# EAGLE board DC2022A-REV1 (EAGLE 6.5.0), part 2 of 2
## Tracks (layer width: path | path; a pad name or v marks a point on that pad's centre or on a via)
+3V3  (via drill 0.25)
  Top 0.203: R23.1 46.14,5.12 45.85,4.83 44.07,4.83 44.07,7.49 43.84,7.47 R16.R1_2 | U6.8 44.03,12.99 44.07,12.95 v43.18,12.95 | 50.93,11.81 U9.18 | R17.1 56.13,7.87 56.13,7.37 55.88,7.11 54.48,7.11 54.23,7.37 54.23,10.67 53.59,11.3 53.59,12.19 | C18.2 27.29,22.25
  Top 0.305: U6.8 44.32,12.95 44.32,11.94 44.3,11.92 44,11.92 C22.1 R16.R4_2 | U4.12 U4.11 29.41,22.42 29.34,22.35 v28.45,22.35 28.45,21.84 C18.2
  Top 0.406: R16.R1_2 R16.R2_2 R16.R3_2 R16.R4_2 | 50.93,11.81 51.31,12.19 53.59,12.19 53.59,12.83 v53.85,13.08 | v28.45,22.35 28.45,22.28 | R15.R1_2 R15.R2_2 R15.R3_2 R15.R4_2 41.62,18.2 41.36,18.2 41.27,18.29 v41.27,19.05
  Route15 0.406: v53.85,13.08 53.85,12.7 53.47,12.32 52.32,12.32 51.94,11.94 45.31,11.94 U6.8 43.22,12.99 v43.18,12.95
  Bottom 0.203: R39.1 R37.1 53.17,15.28 53.85,14.61 v53.85,13.08 | R44.1 23.07,29.21
  Bottom 0.406: v43.18,12.95 43.18,13.59 41.53,15.24 40.83,15.24 R38.R1_2 R38.R2_2 R38.R3_2 R38.R4_2 40.73,18.92 | U12.5 19.81,27.05 19.56,27.3 19.56,29.21 C50.1 23.07,29.21 | 40.73,18.92 40.73,20.23 40.26,20.57 36.83,20.57 35.81,19.56 35.69,19.43 29.97,19.43 29.46,19.94 23.11,19.94 22.35,20.7 22.35,22.1 23.16,22.1 | v41.27,19.05 40.85,19.05 40.73,18.92 | R42.2 23.33,23.91 | 24.38,22.1 28.45,22.1 v28.45,22.35 | R42.2 23.37,24 | 24.38,22.1 24.38,28.83 24.26,28.96 23.41,28.96 R44.1 | 23.16,22.1 23.24,22.1 | 23.24,22.1 23.2,22.19 | 23.2,22.19 23.2,23.88 R42.2 | 23.24,22.1 24.38,22.1 | 23.16,22.1 23.2,22.19
+12V
  Route15 1.016: JP2.14 JP2.13
  pour Top (no thermals): 48.13,30.3 48.13,32.77 57.15,32.77 58.17,33.78 60.58,33.78 61.85,32.64 61.85,30.23 60.33,28.7 53.09,28.7 53.09,29.59 52.32,30.35 50.04,30.35
  pour Bottom (no thermals): 55.12,26.42 55.12,36.45 55.75,37.08 55.75,41.78 56.13,42.16 57.91,42.16 58.29,41.78 58.29,34.29 58.67,33.91 60.58,33.91 61.72,32.89 61.72,30.1 60.07,28.45 60.07,21.08 57.53,18.54 57.53,3.81 57.02,3.3 54.86,3.3 54.86,23.88 57.15,23.88 57.15,26.42
A0_MUX  (via drill 0.25)
  Top 0.203: U9.3 47.88,8.76 47.45,8.38 47.3,8.38 v47.3,8.46 47.3,8.41 47.27,8.38 46.84,8.38 | 46.84,8.38 R16.R2_1 46.59,8.36 46.61,8.38 46.84,8.38
  Bottom 0.203: v47.3,8.46 47.3,8.41 47.27,8.38 46.48,8.38 45.97,7.87 JP3.6
A1_MUX  (via drill 0.25)
  Top 0.203: U9.2 48.67,9.27 47.93,9.27 47.78,9.16 R16.R3_1 46.12,9.16 46.1,9.14 47.3,9.14 | 47.3,9.14 47.4,9.16 | 47.3,9.14 v47.3,9.45 47.3,9.27
  Bottom 0.203: v47.3,9.45 46.41,9.45 46.1,9.14 JP3.7
A2_MUX  (via drill 0.25)
  Top 0.203: 47.3,10.16 48.39,10.16 48.39,9.78 48.64,9.78 U9.1 | R16.R4_1 46.44,10.12 46.48,10.16 47.3,10.16 | 47.3,10.16 v47.3,10.54
  Bottom 0.203: v47.3,10.54 45.21,10.54 JP3.8
ALERTB  (via drill 0.25)
  Top 0.203: U4.31 37.16,18.72 37.34,18.54 37.85,18.54 38.35,18.03 38.35,15.37 38.86,14.86 39.62,14.86 | v42.93,16.51 42.93,15.24 42.55,14.86 39.62,14.86 | R15.R4_1 39.62,15.62 39.62,14.86
  Route15 0.203: v30.73,29.97 30.73,29.34 31.11,28.96 32.51,28.96 32.77,29.21 32.77,30.73 33.02,30.99 33.66,30.99 34.16,31.5 39.12,31.5 39.75,30.86 41.91,30.86 42.16,30.61 42.16,30.1 43.05,29.21 v43.05,28.83
  Bottom 0.203: JP1.3 46.55,38.42 46.23,38.1 45.09,38.1 43.56,36.58 43.56,33.78 43.31,33.53 43.31,28.83 | 43.31,28.83 43.31,20.83 44.2,19.94 44.2,16.51 | 44.2,16.51 44.2,14.73 44.7,14.22 44.7,12.19 44.96,11.94 46.99,11.94 48.13,10.79 48.13,8.26 46.48,6.6 46.48,3.78 JP2.3 | TP12.TP 12.06,26.92 12.57,26.42 16.13,26.42 | 44.2,16.51 v42.93,16.51 | U12.1 18.3,26.4 18.29,26.42 16.13,26.42 | 16.13,26.42 16.13,29.72 16.89,30.48 24.89,30.48 25.27,30.1 30.61,30.1 v30.73,29.97 | v43.05,28.83 43.31,28.83
CTRL  (via drill 0.25)
  Top 0.203: C28.1 55.24,10.03 55.63,10.41 57.02,10.41 57.28,10.67 S1.5 | U4.32 37.65,19.38 37.72,19.43 37.97,19.43 38.41,19.87 U4.33 39.37,20.13 | U4.22 U4.23 33.16,18.81 32.77,18.41 30.99,18.41 30.35,17.78 28.57,17.78 v28.57,17.65 | 39.37,20.13 v39.37,19.81 39.37,18.23 R15.R1_1 | 39.37,20.13 41.98,20.13 v43.18,18.92
  Top 0.406: S1.5 S1.2
  Route15 0.203: v43.18,18.92 43.31,18.92 43.81,18.41 43.81,17.02 44.96,15.88 45.97,15.88 48.01,13.84 50.55,13.84 51.94,15.24 53.21,15.24 54.86,13.59 55.5,13.59 57.15,11.94 S1.5
  Bottom 0.203: 42.55,18.92 42.55,27.56 42.04,28.07 42.04,29.59 42.55,30.1 42.55,34.04 42.8,34.29 42.8,37.08 43.43,37.72 43.43,41.15 | JP2.2 44.55,1.65 43.69,1.65 43.43,1.91 43.43,4.83 43.56,4.95 43.56,12.06 43.94,12.45 43.94,13.72 41.78,15.88 41.78,18.41 42.29,18.92 42.55,18.92 | 43.43,41.15 44.55,41.15 JP1.2 | R56.2 43.43,43.56 43.43,41.15 | 42.55,18.92 v43.18,18.92 | v28.57,17.65 28.32,17.65 27.81,18.16 27.81,18.8 28.19,19.18 29.34,19.18 29.59,18.92 35.94,18.92 36.96,19.94 39.37,19.94 v39.37,19.81
CTRL_P
  Bottom 0.203: R56.1 45.68,43.22 45.72,43.18 50.55,43.18 51.54,42.19 51.54,38.38 52.83,37.08 TP6.TP
DACP_CH0  (via drill 0.25)
  Top 0.203: v36.07,29.46 35.94,29.46 35.69,29.21 35.69,28.4 U4.53
  Route15 0.203: v25.02,16.64 26.16,17.78 26.16,28.32 26.8,28.96 v27.18,28.96
  Bottom 0.203: R36.2 17.02,12.45 17.27,12.45 | TP28.1 17.27,14.73 18.16,15.62 24.64,15.62 25.02,16 v25.02,16.64 | v27.18,28.96 26.92,28.7 26.92,24.13 27.43,23.11 33.53,23.11 35.05,24.51 35.05,26.16 35.56,26.54 35.56,29.34 35.69,29.46 v36.07,29.46
  Bottom 0.406: 17.27,12.45 TP28.1
DACP_CH1  (via drill 0.25)
  Top 0.203: TP24.1 32.64,15.24 32.26,15.62 v32.26,17.78 | U4.54 35.16,29.06 35.31,29.21 35.31,29.59 v36.07,30.35
  Route15 0.203: v32.26,17.78 32.64,17.78 33.53,18.67 33.53,23.62 35.05,25.4 35.05,29.34 v36.07,30.35
  Bottom 0.203: R34.2 32.38,12.45 32.64,12.45
  Bottom 0.406: 32.64,12.45 TP24.1
DACP_CH2
  Top 0.203: TP37.1 21.72,31.5 22.1,31.11 32.38,31.11 32.51,31.11 32.77,30.86 32.77,29.84 33.66,28.96 U4.57
  Bottom 0.203: R48.2 21.97,33.91 21.72,33.91
  Bottom 0.406: TP37.1 21.72,33.91
DACP_CH3  (via drill 0.25)
  Top 0.203: U4.58 33.16,28.44 33.15,28.45 33.15,28.91 32.46,29.59 v32.05,29.59
  Route15 0.203: TP33.1 37.08,32.77 36.83,33.02 36.7,33.02 34.42,33.02 34.04,32.64 34.04,32 33.53,31.5 32.89,31.5 32.13,30.73 32.13,29.67 v32.05,29.59
  Bottom 0.203: R46.2 37.34,33.91 37.08,33.91
  Bottom 0.406: TP33.1 37.08,33.91
EESCL
  Top 0.203: 61.98,6.1 61.72,6.35 R20.1 62.53,6.35 | U10.1 62.32,1.59 62.53,1.78 62.53,6.35 | 62.53,6.35 62.53,6.66 63.12,7.24 63.12,8 63.37,8.26 68.17,8.26 68.67,8.76 68.67,10.29 68.23,10.73 66.52,10.73 J2.11 65.59,9.65
EESDA
  Top 0.203: 61.72,3.43 U10.3 61.72,4.83 R24.1 60.83,4.83 60.83,7.06 60.96,7.19 62.46,7.19 62.61,7.34 62.61,8.26 62.99,8.64 67.41,8.64 67.69,8.89 67.69,9.65 J2.12
EEVCC  (via drill 0.25)
  Top 0.203: 63.32,20.77 62.7,20.77 C19.1
  Top 0.254: U5.8 U5.7
  Top 0.406: R24.2 R20.2 59.94,6.35 | U10.4 58.86,3.49 59.18,3.56 | 59.18,4.79 R24.2 | 59.18,3.56 59.05,3.56 | 59.18,4.79 59.18,4.83 | 59.18,3.56 59.18,4.79 | R24.2 59.18,4.83 | 59.18,4.83 v58.8,4.83 | 59.94,6.35 59.86,6.35 | 59.94,6.35 59.94,7.87 C27.1
  Top 0.813: 68.42,37.85 68.4,37.82 68.58,37.82 68.58,22.48 68.45,22.48 68.4,22.55
  Top 1.016: 68.42,37.85 67.41,38.86 64.14,38.86 63.37,39.62 59.31,39.62 58.04,40.89 58.04,42.55 57.66,42.93 51.05,42.93 50.53,42.4 50.53,41.15 JP1.8 | 64.14,22.48 68.45,22.48 | 64.14,22.48 v64.14,21.84 64.14,21.59 63.32,20.77 U5.8 | 64.14,22.48 v64.14,22.99
  Route15 0.406: v52.58,19.56 54.1,19.56 56.39,21.84 v64.14,21.84
  Bottom 0.406: D1.2 53.48,19.8 53.09,19.56 v52.58,19.56
  Bottom 0.813: J2.1 65.52,19.7 65.5,19.68 64.1,19.68 arc60 64.14,19.81 v64.14,21.84 v64.14,22.99
  pour Bottom (no thermals): 49.78,2.92 57.28,2.92 58.04,3.68 58.04,18.29 60.58,20.83 66.39,20.83 66.39,18.92 62.23,18.92 59.82,16.51 59.82,0.76 49.78,0.76
  pour Top (no thermals): 60.2,21.46 63.12,21.46 63.5,21.84 63.5,23.5 64.9,23.5 64.9,21.72 63.37,20.19 60.2,20.19
FAULTB  (via drill 0.25)
  Top 0.203: U4.25 U4.26 34.47,19.38 34.42,19.3 34.42,17.27 34.8,16.89 v34.8,15.24 | TP7.TP 9.27,31.37 10.16,30.48 14.73,30.48 15.37,29.84 15.37,27.94 15.61,27.7 v17.13,27.7
  Route15 0.203: v43.18,19.81 42.8,19.81 42.29,19.3 42.29,16.13 41.66,15.49 35.05,15.49 v34.8,15.24
  Bottom 0.203: JP2.1 44.29,3.72 44.2,3.81 44.2,6.35 44.07,6.48 44.07,11.94 44.32,12.19 44.32,13.97 42.29,16 42.29,17.65 42.67,18.03 43.43,18.03 43.81,18.41 43.81,19.43 43.43,19.81 v43.18,19.81 42.93,19.81 42.93,27.81 42.42,28.32 42.42,29.34 42.93,29.84 42.93,33.78 43.18,34.04 43.18,36.83 44.58,38.23 44.58,39.13 JP1.1 | v17.13,27.7 U12.3 19.05,27.7 19.05,26.16 19.3,25.91 20.7,25.91 20.95,25.65 20.95,25.02 21.84,24.13 21.84,20.32 22.86,19.3 26.04,19.3 29.72,15.62 32.89,15.62 33.78,14.73 34.29,14.73 v34.8,15.24 35.05,15.49 37.34,15.49 38.08,16.24 R38.R2_1
FB_LTC3604
  Top 0.203: 51.73,23.75 R8.2 51.85,24.42 52.07,24.64 52.7,24.64 52.96,24.89 52.96,27.05 52.7,27.3 52.7,28.96 52.3,29.44 U3.11
  Top 0.305: R9.1 C17.1 51.73,23.75 | R8.2 C13.2
GND  (via drill 0.25, 0.25 pad 0.56)
  Top 0.203: v40.77,13.72 v41.78,13.72 | C24.2 v40.77,13.72 | v40.77,13.72 v39.75,13.72 | v40.77,13.72 40.77,12.2 | R22.1 33.62,6.39 33.53,6.1 | v25.4,13.72 v26.42,13.72 | C23.2 v25.4,13.72 | v25.4,13.72 v24.38,13.72 | v25.4,13.72 25.4,12.2 | R21.1 18.25,6.39 18.16,6.1 | v12.57,32.64 v13.59,32.64 | v13.59,32.64 C9.2 | v13.59,32.64 v14.61,32.64 | v13.59,32.64 13.59,34.16 | R3.1 20.74,39.97 20.83,40.26 | v27.94,32.64 v28.96,32.64 | v28.96,32.64 C10.2 | v28.96,32.64 v29.97,32.64 | v28.96,32.64 28.96,34.16 | R4.1 36.11,39.97 36.2,40.26
  Top 0.305: LED3.N 45.6,17.03 45.85,17.27 45.85,19.43 46.1,19.68 v46.61,19.68
  Top 0.406: 33.53,6.1 33.66,6.22 33.91,6.22 | v34.67,6.22 33.62,6.22 R22.1 | 18.16,6.1 18.29,6.22 18.54,6.22 | v19.3,6.22 18.25,6.22 R21.1 | 20.83,40.26 20.7,40.13 20.45,40.13 | v19.68,40.13 20.74,40.13 R3.1 | 36.2,40.26 36.07,40.13 35.81,40.13 | v35.05,40.13 36.11,40.13 R4.1
  Bottom 0.203: 42.16,3.03 Q5.2 | 42.16,3.03 42.16,3.05 | v42.16,2.29 42.16,3.03 | 26.8,3.03 Q6.2 | 26.8,3.03 26.8,3.05 | v26.8,2.29 26.8,3.03 | Q9.2 12.19,43.32 | 12.19,43.32 12.19,43.31 | 12.19,43.32 v12.19,44.07 | Q8.2 27.56,43.32 | 27.56,43.32 27.56,43.31 | 27.56,43.32 v27.56,44.07 | 46.86,19.81 47.12,20.32
  Bottom 0.406: C36.1 C37.2 | C38.1 C39.2 | C61.1 C60.2 | C59.1 C58.2 | 64.23,7.34 64.23,17.78 65.64,17.78 J2.3
  other vias: 29.97,3.05 28.45,3.05 29.59,7.37 14.61,3.05 13.08,3.05 14.22,7.37 24.38,43.31 25.91,43.31 24.77,38.99 39.75,43.31 41.27,43.31 40.13,38.99 50.93,8.76 48.26,14.61 52.7,14.22 49.78,29.21 65.53,7.49 60.07,2.54 57.78,4.57 44.45,25.02 44.45,26.04 55.75,18.29 63.12,18.03 53.85,25.15 54.99,25.15 56.13,25.15 35.69,21.97 25.02,18.67 32,21.97 30.23,17.02 32,25.65 35.69,25.65 41.4,28.57
  pour Top (no thermals): 38.73,14.35 42.29,14.35 42.29,11.05 37.47,11.05 36.83,11.68 36.83,13.34 37.47,13.34 37.47,11.94 37.72,11.68 38.48,11.68 38.73,11.94
  pour Bottom (no thermals): 38.73,14.35 42.29,14.35 42.29,11.18 39.12,11.18 38.73,11.56
  pour Bottom (no thermals): 34.04,5.08 31.88,5.08 30.73,3.94 30.73,2.29 27.56,2.29 27.56,9.4 31.62,9.4 32,9.78 33.15,9.78 33.53,10.16 33.53,11.3 35.43,11.3 35.43,9.78 35.05,9.4 35.05,6.1
  pour Top (no thermals): 30.1,8.89 30.86,8.89 31.11,8.64 31.11,2.29 27.56,2.29 27.56,8.51 29.08,8.51 29.21,8.64 29.21,9.91 28.96,10.16 28.32,10.16 28.32,13.34 29.34,13.34 29.34,12.06 29.59,11.81 29.59,9.4
  pour Top (no thermals): 23.37,14.35 26.92,14.35 26.92,11.05 22.1,11.05 21.46,11.68 21.46,13.34 22.1,13.34 22.1,11.94 22.35,11.68 23.11,11.68 23.37,11.94
  pour Bottom (no thermals): 23.37,14.35 26.92,14.35 26.92,11.18 23.75,11.18 23.37,11.56
  pour Bottom (no thermals): 18.67,5.08 16.51,5.08 15.37,3.94 15.37,2.29 11.94,2.29 11.94,9.4 16.26,9.4 16.64,9.78 17.78,9.78 18.16,10.16 18.16,11.3 20.07,11.3 20.07,9.78 19.68,9.4 19.68,6.1
  pour Top (no thermals): 14.73,8.89 15.49,8.89 15.75,8.64 15.75,2.29 11.94,2.29 11.94,8.51 13.72,8.51 13.84,8.64 13.84,9.91 13.59,10.16 12.95,10.16 12.95,13.34 13.97,13.34 13.97,12.06 14.22,11.81 14.22,9.4
  pour Top (no thermals): 15.62,32 11.81,32 11.81,35.31 16.89,35.31 17.53,34.67 17.53,33.02 16.89,33.02 16.89,34.42 16.64,34.67 15.88,34.67 15.62,34.42
  pour Bottom (no thermals): 15.62,32 12.06,32 12.06,35.18 15.24,35.18 15.62,34.8
  pour Bottom (no thermals): 20.32,41.27 22.48,41.27 23.62,42.42 23.62,44.07 26.8,44.07 26.8,36.96 22.73,36.96 22.35,36.58 21.21,36.58 20.83,36.2 20.83,35.05 18.92,35.05 18.92,36.58 19.3,36.96 19.3,40.26
  pour Top (no thermals): 24.26,37.47 23.5,37.47 23.24,37.72 23.24,44.07 26.8,44.07 26.8,37.85 25.27,37.85 25.15,37.72 25.15,36.45 25.4,36.2 26.04,36.2 26.04,33.02 25.02,33.02 25.02,34.29 24.77,34.54 24.77,36.96
  pour Top (no thermals): 30.99,32 27.43,32 27.43,35.31 32.26,35.31 32.89,34.67 32.89,33.02 32.26,33.02 32.26,34.42 32,34.67 31.24,34.67 30.99,34.42
  pour Bottom (no thermals): 30.99,32 27.43,32 27.43,35.18 30.61,35.18 30.99,34.8
  pour Bottom (no thermals): 35.69,41.27 37.85,41.27 38.99,42.42 38.99,44.07 42.16,44.07 42.16,36.96 38.1,36.96 37.72,36.58 36.58,36.58 36.2,36.2 36.2,35.05 34.29,35.05 34.29,36.58 34.67,36.96 34.67,40.26
  pour Top (no thermals): 39.62,37.47 38.86,37.47 38.61,37.72 38.61,44.07 42.16,44.07 42.16,37.85 40.64,37.85 40.51,37.72 40.51,36.45 40.77,36.2 41.4,36.2 41.4,33.02 40.39,33.02 40.39,34.29 40.13,34.54 40.13,36.96
  pour Top (no thermals): 42.29,14.35 11.81,14.35 11.81,0.76 1.78,0.76 0.89,1.65 0.89,45.59 12.57,45.59 12.57,43.94 11.81,43.18 11.81,40.01 11.56,39.75 11.56,35.56 11.81,35.31 11.81,32 43.43,32 43.43,26.42 44.58,26.42 44.83,26.16 44.83,19.18 65.41,19.18 65.41,22.99 68.07,22.99 68.07,27.56 62.36,27.56 62.36,32.77 60.71,34.29 57.91,34.29 56.9,33.27 47.62,33.27 47.62,32.38 43.43,32.38 43.43,32.13 42.29,32.13 42.29,45.59 68.93,45.59 68.93,0.76 42.29,0.76 42.29,6.35 42.8,6.35 42.8,11.05 42.29,11.05
  pour Route2 (no thermals): 0.89,45.59 0.89,3.05 3.17,0.76 68.93,0.76 68.93,45.59
  pour Bottom (no thermals): 11.81,32 42.16,32 42.16,45.59 68.93,45.59 68.93,0.76 60.33,0.76 60.33,16.38 62.36,18.41 66.77,18.41 66.8,21.21 64.9,21.21 64.9,23.37 68.07,23.37 68.07,27.56 63.75,27.56 63.75,21.34 60.58,21.34 60.58,28.19 62.23,29.84 62.23,33.15 60.83,34.42 58.93,34.42 58.8,34.54 58.8,41.91 58.04,42.67 56.01,42.67 55.37,42.04 55.37,37.34 54.74,36.7 54.74,25.91 56.64,25.91 56.64,24.38 54.36,24.38 54.36,3.3 49.4,3.3 49.4,0.76 42.42,0.76 42.42,8.13 42.67,8.38 42.67,10.29 42.42,10.54 42.42,14.35 11.81,14.35 11.81,0.76 0.89,0.76 0.89,45.59 11.81,45.59
  pour Top (no thermals): 49.02,29.84 52.2,29.84 52.7,29.34 52.7,28.19 60.58,28.19 62.36,29.97 62.36,27.56 56.52,27.56 56.52,24.26 61.34,24.26 62.1,23.5 62.99,23.5 62.99,21.97 62.87,21.84 49.78,21.84 49.78,25.02 49.02,25.02
  pour Top: 30.48,26.67 30.48,20.95 36.83,20.95 36.83,26.67
IBV_AUX  (via drill 0.25)
  Top 0.203: C13.1 48.68,24.42 48.84,24.59 50.75,24.59 51.31,25.15 51.31,26.04 50.42,26.92 50.42,27.34 U3.8 | 46.23,27.51 46.23,25.02 | U5.1 55.47,20.77 C20.1 | v51.69,21.21 51.69,21.03 52.45,20.77
  Top 0.254: U5.1 U5.2
  Top 0.406: C13.1 48.55,23.75 R9.2 46.99,22.23 46.35,22.23 46.35,22.99 C15.1 46.23,22.99 46.23,27.51 L3.2
  Top 1.016: 51.38,20.77 52.45,20.77 U5.1 | 46.99,22.23 46.99,21.72 48.19,20.77 51.38,20.77 | R11.2 51.47,20.73 51.44,20.83 51.38,20.77
  Bottom 0.406: D1.1 51.7,21.1 v51.69,21.21
  pour Top (no thermals): 45.34,19.81 45.34,26.42 44.96,26.8 43.94,26.8 43.94,28.32 46.1,28.32 46.61,27.81 46.61,24.51 49.28,24.51 49.28,21.46 57.66,21.46 57.66,19.94 57.53,19.81
IIN_SNSM  (via drill 0.25)
  Top 0.203: v64.9,27.05 64.52,26.67 NB6.2 | v33.4,30.35 33.4,29.97 34.16,29.21 U4.56
  Route15 0.203: v33.4,30.35 33.66,30.35 34.42,31.11 38.73,31.11 40.26,29.59 41.91,29.59 42.42,29.08 42.42,28.45 43.43,27.43 62.99,27.43 63.25,27.69 64.26,27.69 v64.9,27.05
IIN_SNSP  (via drill 0.25)
  Top 0.203: v63.63,27.05 64.01,26.67 NB5.2 | v35.18,30.35 35.18,30.1 34.66,29.58 U4.55 | U4.9 28.57,23.63 v28.37,23.88
  Route15 0.203: v63.63,27.05 43.18,27.05 42.04,28.19 42.04,28.83 41.66,29.21 39.88,29.21 38.73,30.35 v36.96,30.35
  Bottom 0.203: v36.96,30.35 36.96,30.73 36.7,30.99 35.43,30.99 35.18,30.73 v35.18,30.35 34.67,29.84 34.67,27.3 31.11,23.88 v28.37,23.88
INTVCC_LTC3604  (via drill 0.25)
  Top 0.203: v50.55,25.73 50.55,26.16 49.91,26.8 49.91,27.33 U3.7 | U3.1 47.27,29.94 47.24,29.97 v47.24,30.61 | U3.10 52.08,28.94 52.2,28.83 v52.2,25.4
  Bottom 0.203: C51.1 53.47,27.22 53.43,27.18 52.2,27.18 | 50.55,27.18 v50.55,25.73 | 50.55,27.18 47.37,27.18 47.24,27.3 v47.24,30.61 | 50.55,27.18 52.2,27.18 | 52.2,27.18 v52.2,25.4
ISNSN_CH0  (via drill 0.25)
  Top 0.203: C30.1 14.86,5.97 14.86,6.6 15.37,7.11 v15.37,8.26 15.37,8.89 14.61,9.65 14.61,12.06 14.35,12.32 14.35,13.46 13.97,13.84 TP30.1 13.97,14.22 15.37,15.62 22.73,15.62 23.11,16 v23.11,21.34 | v41.02,25.27 40.26,25.27 39.62,24.64 38.61,24.64 38.6,24.63 U4.42
  Bottom 0.203: R32.R4_1 15.27,9.37 15.37,9.27 v15.37,8.26 | v23.11,21.34 24.26,21.34 24.64,20.95 29.84,20.95 30.48,20.32 35.18,20.32 36.32,21.46 39.75,21.46 40.13,21.84 40.13,25.15 40.26,25.27 v41.02,25.27
ISNSN_CH1  (via drill 0.25)
  Top 0.203: C31.1 30.23,5.97 30.23,6.6 30.73,7.11 v30.73,8.26 30.73,8.89 29.97,9.65 29.97,12.06 29.72,12.32 29.72,13.46 29.34,13.84 TP26.1 v29.34,17.02 | v41.02,27.3 39.37,25.65 38.44,25.65 U4.44
  Route15 0.203: v29.34,17.02 29.34,17.4 29.59,17.65 31.37,17.65 31.88,17.14 32.64,17.14 34.04,18.54 34.04,23.5 34.92,24.38 39.75,24.38 40.01,24.64 40.01,26.8 40.51,27.3 v41.02,27.3
  Bottom 0.203: R31.R4_1 30.63,9.37 30.73,9.27 v30.73,8.26
ISNSN_CH2  (via drill 0.25)
  Top 0.203: TP35.1 24.89,32.64 24.64,32.89 24.64,34.04 24.38,34.29 24.38,36.7 23.62,37.47 v23.62,38.1 23.62,39.24 24.13,39.75 24.13,40.39 C5.1 | v40.51,30.23 40.39,30.23 40.39,28.32 39.88,27.81 39.88,27.43 39.07,26.63 U4.46
  Route15 0.203: TP35.1 24.89,32
  Bottom 0.203: R51.R4_1 23.72,36.98 23.62,37.08 v23.62,38.1 | v40.51,30.23 38.99,30.23 37.85,31.37 34.29,31.37 34.04,31.11 25.53,31.11 24.89,31.75 TP35.1
ISNSN_CH3  (via drill 0.25)
  Top 0.203: C6.1 39.5,40.39 39.5,39.75 38.99,39.24 v38.99,38.1 38.99,37.47 39.75,36.7 39.75,34.29 40.01,34.04 40.01,32.89 40.39,32.51 TP31.1 40.39,31.88 39.5,30.99 39.5,28.7 38.99,28.19 38.99,27.94 38.73,27.69 38.35,27.69 U4.48
  Bottom 0.203: R50.R4_1 39.09,36.98 38.99,37.08 v38.99,38.1
ISNSP_CH0  (via drill 0.25)
  Top 0.203: C32.1 15.37,4.45 15.37,4.95 15.75,5.33 15.75,6.73 16.13,7.11 16.13,8.76 14.99,9.91 14.99,12.32 14.73,12.57 14.73,13.46 TP29.1 15.37,14.48 16.13,15.24 23.11,15.24 23.62,15.75 23.62,20.7 v23.88,20.7 | U4.41 40.77,24.13 v41.02,24.38
  Bottom 0.203: TP29.1 15.37,13.72 14.61,12.95 14.61,12 R32.R1_1 | v23.88,20.7 24,20.57 29.59,20.57 30.23,19.94 35.43,19.94 35.56,20.07 36.58,21.08 40.13,21.08 40.51,21.46 40.51,24.26 40.64,24.38 40.77,24.38 v41.02,24.38
ISNSP_CH1  (via drill 0.25)
  Top 0.203: C34.1 30.73,4.45 30.73,4.95 31.11,5.33 31.11,6.73 31.5,7.11 31.5,8.76 30.35,9.91 30.35,12.32 30.1,12.57 30.1,13.46 TP25.1 30.73,15.24 31.11,15.62 v31.11,17.02 | v41.02,26.29 40.64,26.29 39.5,25.15 38.43,25.15 U4.43
  Route15 0.203: v31.11,17.02 31.11,16.76 32.89,16.76 34.54,18.41 34.54,23.37 35.18,24 40.13,24 40.39,24.26 40.39,26.04 40.64,26.29 v41.02,26.29
  Bottom 0.203: TP25.1 30.73,13.72 29.97,12.95 29.97,12 R31.R1_1
ISNSP_CH2  (via drill 0.25)
  Top 0.203: TP36.1 24.26,32.89 24.26,33.78 24,34.04 24,36.45 22.86,37.59 22.86,39.24 23.24,39.62 23.24,41.02 23.62,41.4 23.62,41.91 C2.1 | U4.45 39.21,26.13 40.26,27.18 40.26,27.56 40.77,28.07 40.77,29.21 41.4,29.84 v41.4,30.23
  Route15 0.203: v33.15,32.13 33.15,32.77 33.78,33.4 37.34,33.4 37.72,33.4 37.97,33.15 v37.97,32.77
  Bottom 0.203: TP36.1 23.62,32.77 23.88,33.02 24.38,33.02 | 24.38,33.02 24.38,34.35 R51.R1_1 | v41.4,30.23 41.4,30.61 41.15,30.86 40.89,30.86 39.12,30.86 37.97,32 v37.97,32.77 | 24.38,33.02 25.4,33.02 25.65,32.77 25.65,31.75 25.91,31.5 32.89,31.5 33.15,31.75 v33.15,32.13
ISNSP_CH3  (via drill 0.25)
  Top 0.203: TP32.1 39.62,32.89 39.62,33.78 39.37,34.04 39.37,36.45 38.23,37.59 38.23,39.24 38.61,39.62 38.61,41.02 38.99,41.4 38.99,41.91 C4.1 | U4.47 38.94,27.13 39.5,27.69 39.5,28.07 39.88,28.45 39.88,30.61 40.77,31.5 v41.15,31.5
  Bottom 0.203: R50.R1_1 39.75,34.35 39.75,33.02 TP32.1 38.99,31.75 39.24,31.5 v41.15,31.5
ITH_LTC3604  (via drill 0.25)
  Top 0.203: U3.12 52.17,29.94 52.32,30.1 v52.32,30.86
  Bottom 0.203: v52.32,30.86 52.07,30.86 52.07,28.83 51.05,28.83 | 51.02,28.83 R45.2 51.05,28.83 | C52.1 48.77,28.57 51.05,28.57 51.05,28.83
N$1
  Bottom 0.406: D1.3 51.31,20.45 50.55,21.21 C46.1 49.66,21.34 49.02,21.97 49.02,24.26 49.22,24.45 U11.4
N$3  (via drill 0.25)
  Top 0.203: v22.1,27.94 LED1.P
  Bottom 0.203: v22.1,27.94 22.1,27.43 22.31,27.22 23.33,27.22 23.37,27.18 R44.2
N$4  (via drill 0.25)
  Top 0.203: U9.16 52.7,11.01 v52.7,11.43
  Route15 0.203: v52.7,11.43 44.96,11.43 44.07,12.32 31.5,12.32 31.24,12.06 30.73,12.06 29.72,13.08 16.76,13.08 v16.38,13.46
  Bottom 0.203: v16.38,13.46 16.38,22.48 16,22.86 R41.1
N$9
  Top 0.406: P4.P 42.16,3.3 42.16,5.59 41.4,5.59 R19.1
N$10  (via drill 0.25)
  Top 0.203: v38.86,2.67 39.24,3.05 39.76,3.05 P4.N
  Bottom 0.203: v38.86,2.67 40.13,2.67 40.13,3.68 Q5.3
N$11
  Bottom 0.203: 28.09,9.37 28.07,9.4 28.23,9.4 | C37.1 28.45,6.86 28.19,7.11 28.19,9.27 28.09,9.37 | 28.07,10.18 R31.R3_2 | 28.09,9.37 R31.R4_2
  Bottom 0.406: 28.07,9.4 28.07,10.18
N$12
  Bottom 0.203: C36.2 29.97,5.59 30.35,5.59 30.35,7.62 29.97,8 29.97,8.64 29.08,8.64 29.08,10.92 28.96,11.05 28,11.05 R31.R2_2
  Bottom 0.406: R31.R2_2 R31.R1_2
N$13  (via drill 0.25)
  Top 0.203: NB10.1 31.5,10.79 v31.5,10.41
  Bottom 0.203: R31.R3_1 31.35,10.27 v31.5,10.41
N$14
  Top 0.406: P3.P 26.8,3.3 26.8,5.59 26.04,5.59 R18.1
N$15  (via drill 0.25)
  Top 0.203: v23.5,2.67 23.88,3.05 24.4,3.05 P3.N
  Bottom 0.203: v23.5,2.67 24.77,2.67 24.77,3.68 Q6.3
N$16
  Bottom 0.203: 12.72,9.37 12.7,9.4 12.87,9.4 | C39.1 13.08,6.86 12.83,7.11 12.83,9.27 12.72,9.37 | 12.7,10.18 R32.R3_2 | 12.72,9.37 R32.R4_2
  Bottom 0.406: 12.7,9.4 12.7,10.18
N$17
  Bottom 0.203: C38.2 14.61,5.59 14.99,5.59 14.99,7.62 14.61,8 14.61,8.64 13.72,8.64 13.72,10.92 13.59,11.05 12.63,11.05 R32.R2_2
  Bottom 0.406: R32.R2_2 R32.R1_2
N$18  (via drill 0.25)
  Top 0.203: NB9.1 16.13,10.79 v16.13,10.41
  Bottom 0.203: R32.R3_1 15.98,10.27 v16.13,10.41
N$19
  Top 0.406: P1.P 12.19,43.05 12.19,40.77 12.95,40.77 R5.1
N$20  (via drill 0.25)
  Top 0.203: v15.49,43.69 15.11,43.31 14.59,43.31 P1.N
  Bottom 0.203: v15.49,43.69 14.22,43.69 14.22,42.67 Q9.3
N$21
  Bottom 0.203: 26.26,36.98 26.29,36.96 26.12,36.96 | C60.1 25.91,39.5 26.16,39.24 26.16,37.08 26.26,36.98 | 26.29,36.17 R51.R3_2 | R51.R4_2 26.26,36.98
  Bottom 0.406: 26.29,36.96 26.29,36.17
N$22
  Bottom 0.203: C61.2 24.38,40.77 24,40.77 24,38.73 24.38,38.35 24.38,37.72 25.27,37.72 25.27,35.43 25.4,35.31 26.36,35.31 R51.R2_2
  Bottom 0.406: R51.R2_2 R51.R1_2
N$23  (via drill 0.25)
  Top 0.203: NB1.1 22.86,35.56 v22.86,35.94
  Bottom 0.203: R51.R3_1 23.01,36.09 v22.86,35.94
N$24
  Top 0.406: P2.P 27.56,43.05 27.56,40.77 28.32,40.77 R6.1
N$25  (via drill 0.25)
  Top 0.203: v30.86,43.69 30.48,43.31 29.96,43.31 P2.N
  Bottom 0.203: v30.86,43.69 29.59,43.69 29.59,42.67 Q8.3
N$26
  Bottom 0.203: R50.R4_2 41.66,36.96 41.49,36.96 | C58.1 41.27,39.5 41.53,39.24 41.53,37.08 R50.R4_2 | 41.66,36.17 R50.R3_2 | R50.R4_2
  Bottom 0.406: 41.66,36.96 41.66,36.17
N$27
  Bottom 0.203: C59.2 39.75,40.77 39.37,40.77 39.37,38.73 39.75,38.35 39.75,37.72 40.64,37.72 40.64,35.43 40.77,35.31 41.72,35.31 R50.R2_2
  Bottom 0.406: R50.R2_2 R50.R1_2
N$28  (via drill 0.25)
  Top 0.203: NB2.1 38.23,35.56 v38.23,35.94
  Bottom 0.203: R50.R3_1 38.37,36.09 v38.23,35.94
N$48
  Top 0.203: U4.40 41.45,23.63 C16.1
N$49
  Top 0.203: U4.38 39.14,22.63 39.24,22.73 40.01,22.73 40.11,22.63 40.89,21.84 41.19,21.84 C16.2
N$52
  Top 0.203: U4.13 U4.14 28.36,21.13 27.81,20.57 27.56,20.57 27.3,20.49 C21.2
N$57  (via drill 0.25)
  Top 0.203: v22.1,25.65 LED2.P
  Bottom 0.203: v22.1,25.65 23.37,25.65 R42.1
N$58  (via drill 0.25)
  Top 0.203: LED1.N 24.64,27.18 22.35,27.18 22.1,26.92 v22.1,26.54
  Bottom 0.203: v22.1,26.54 21.72,26.54 21.34,26.92 21.34,27.43 21.08,27.69 20.57,27.69 20.57,27.74 U12.4
N$60  (via drill 0.25)
  Top 0.203: LED2.N 24.13,25.65 23.88,25.4 23.88,24.77 v22.1,24.77
  Bottom 0.203: v22.1,24.77 21.84,24.77 21.46,25.15 21.46,26.04 21.08,26.42 20.55,26.42 U12.6
N$61
  Bottom 0.203: 51.05,31.46 C53.1
  Bottom 0.406: R45.1 51.05,31.46
N$63
  Top 0.305: R10.1 44.45,20.7 LED3.P
N$64  (via drill 0.25)
  Top 0.203: R14.2 60.2,18.33 60.2,18.92 59.69,19.43 v59.31,19.43 59.18,19.43 U5.5
  Route15 0.203: v59.31,19.43 54.74,19.43 54.23,18.92 52.2,18.92 51.94,19.18 51.94,19.94 52.32,20.32 53.47,20.32 54.61,21.46 v54.61,22.35
  Bottom 0.203: v54.61,22.35 R40.1
N$66
  Top 0.203: U9.4 48.09,8.29 47.5,7.7 47.5,7.24 46.99,6.73 46.99,5.08 47.24,4.83 48.51,4.83 48.77,5.08 50.04,5.08 50.34,4.78 50.62,4.78 50.9,4.65 51.38,4.65 52.7,5.97 53.85,5.97 54.48,5.33 56.81,5.33 C29.1 56.81,6.39 56.77,6.48 | 58.25,7.75 R17.2
  Top 0.254: 56.77,6.48 57.28,6.48 57.28,6.99 57.91,7.62 57.91,7.75 58.25,7.75
N$68
  Top 0.203: U5.4 58.68,19.56 58.67,18.29 58.67,18.33 R13.2
N$69
  Top 0.203: U5.6 59.68,20.08 60.07,19.68 60.71,19.68 61.09,19.3 61.09,17.4 60.96,17.27 57.91,17.27 57.78,17.4 57.78,19.18 | 58.17,20.76 U5.3 58.18,19.44 57.91,19.18 57.78,19.18 | 57.78,19.18 53.59,19.18 53.34,18.92 53.34,18.41 52.96,18.41 52.96,18.33 R12.2 53,18.29 | R11.1 51.44,18.29
  Top 0.406: 51.44,18.29 R12.2
N$70
  Top 0.203: 49.17,25.63 49.17,25.59 C12.2 49.15,25.49 49.15,25.65 | 49.15,25.65 49.28,25.65 | 49.15,25.65 49.15,26.7 49.45,27 U3.6
N$74  (via drill 0.25)
  Top 0.203: R23.2 47.88,5.84 47.88,5.46 51.05,5.46 | 51.05,5.46 v51.05,5.33 | 51.05,5.46 51.31,5.46 51.44,5.59 U9.9 | U6.1 50.33,12.99 v50.55,13.21
  Bottom 0.203: v50.55,13.21 50.8,12.95 50.8,10.16 51.69,9.27 51.69,5.71 51.44,5.46 51.05,5.46 v51.05,5.33
RESETB  (via drill 0.25)
  Top 0.203: U4.24 33.66,19.31 33.66,19.3 33.66,17.53 33.66,15.75 v33.91,15.49 | SW1.SW1 13.59,28.96 v13.59,27.43
  Route15 0.203: v46.61,16.38 45.21,16.38 44.2,17.4 44.2,18.67 43.94,18.92 43.94,19.94 43.43,20.45 42.67,20.45 41.91,19.68 41.91,16.38 41.53,16 34.29,16 33.91,15.62 | v13.59,27.43 13.59,25.15 14.48,24.26 14.48,23.75 13.84,23.11 8.13,23.11 7.11,22.1 7.11,18.29 9.78,15.62 33.91,15.62 | 33.91,15.62 v33.91,15.49
  Bottom 0.203: 46.61,15.88 46.74,15.88 46.86,15.75 49.66,15.75 50.55,16.64 50.55,17.27 50.8,17.53 52.07,17.53 52.32,17.27 52.32,15.49 51.56,14.73 49.78,14.73 49.78,12.7 50.16,12.32 50.16,5.08 50.53,4.71 50.55,4.69 JP2.7 | 46.61,15.88 45.97,15.88 45.72,16.13 45.72,19.81 46.1,20.19 46.1,31.88 47.37,31.88 49.66,34.16 49.66,37.34 50.55,38.23 JP1.7 | v46.61,16.38 46.61,15.88 | R38.R3_1 38.12,17.04 37.08,16 34.29,16 33.91,15.62 v33.91,15.49
  Bottom 0.406: C62.2 13.59,28.74 v13.59,27.43
RUN_CH0  (via drill 0.25)
  Top 0.203: U7.1 22.68,14.03 22.61,14.1 TP16.1 | U4.3 28.75,26.63 28.19,27.18 v28.07,27.18
  Route15 0.203: v27.18,16.64 27.18,16.76 26.92,17.02 26.92,26.54 27.56,27.18 v28.07,27.18
  Bottom 0.203: R30.1 26.5,7.58 27.18,8.26 27.18,10.41 26.8,10.79 23.37,10.79 22.48,11.68 TP16.1 23.24,14.86 26.54,14.86 27.18,15.49 v27.18,16.64
  Bottom 0.406: Q6.1 26.76,4.33 26.8,4.45 26.8,5.97 R30.1
RUN_CH1  (via drill 0.25)
  Top 0.203: U8.1 38.04,14.03 37.97,14.1 TP18.1 37.34,14.61 v37.34,17.53 | U4.4 28.1,26.13 v28.07,26.29
  Route15 0.203: v28.07,26.29 27.81,26.29 27.3,25.78 27.3,17.53 28.45,16.38 33.15,16.38 33.78,17.02 36.07,17.02 36.58,17.53 v37.34,17.53
  Bottom 0.203: R29.1 41.87,7.58 42.55,8.26 42.55,10.41 42.16,10.79 38.73,10.79 37.85,11.68 TP18.1
  Bottom 0.406: Q5.1 42.12,4.33 42.16,4.45 42.16,5.97 R29.1
RUN_CH2
  Top 0.203: U1.1 16.31,32.33 16.38,32.26 TP8.1 17.27,31.5 20.45,31.5 21.72,30.23 26.16,30.23 26.42,29.97 26.42,28.7 26.8,28.32 27.18,28.32 27.33,28.17 27.33,25.75 27.43,25.65 29.34,25.65 U4.5
  Bottom 0.203: R53.1 12.48,38.77 11.81,38.1 11.81,35.94 12.19,35.56 15.62,35.56 16.51,34.67 TP8.1
  Bottom 0.406: Q9.1 12.23,42.02 12.19,41.91 12.19,40.39 R53.1
RUN_CH3  (via drill 0.25)
  Top 0.203: U2.1 31.68,32.33 31.75,32.26 TP10.1 | U4.6 28.43,25.13 28.32,25.02 v28.32,24.77
  Route15 0.203: v28.32,24.77 29.34,24.77 29.59,25.02 29.59,30.73 31.11,32.26 TP10.1
  Bottom 0.203: R52.1 27.85,38.77 27.18,38.1 27.18,35.94 27.56,35.56 30.99,35.56 31.88,34.67 TP10.1
  Bottom 0.406: Q8.1 27.6,42.02 27.56,41.91 27.56,40.39 R52.1
SCL  (via drill 0.25)
  Top 0.203: 36.66,18.2 36.7,18.16 37.59,18.16 37.97,17.78 37.97,15.11 38.61,14.48 42.93,14.48 43.43,14.99 43.43,15.49 44.96,15.49 45.34,15.11 45.34,14.61 45.72,14.22 46.23,14.22 46.61,13.84 46.61,13.34 47.12,12.83 47.75,12.83 48.51,13.59 49.36,13.59 U6.2 | 36.66,18.2 36.66,16.68 v36.7,16.64 | 36.66,18.2 U4.30
  Route15 0.203: v36.7,16.64 36.7,16.51 33.91,16.51 33.4,16 10.29,16 9.27,17.02 TP13.TP
  Bottom 0.203: R38.R4_1 38.76,17.93 38.73,17.91 38.73,18.03 38.61,18.16 36.96,18.16 36.7,17.91 v36.7,16.64
SCL_IN  (via drill 0.25)
  Top 0.203: U6.3 49.1,14.22 51.56,14.22 | J2.4 67.52,17.64 66.62,16.74 64.84,16.74 64.23,16.13 51.56,16.13 51.56,15.62 | 51.56,14.22 51.56,13.08 50.42,12.06 50.42,11.02 U9.19 | v50.67,15.62 51.56,15.62 | 51.56,15.62 51.56,14.22
  Bottom 0.203: 49.28,15.24 46.74,15.24 46.48,15.49 45.59,15.49 45.34,15.75 45.34,20.19 45.72,20.57 45.72,32.26 47.12,32.26 49.15,34.29 49.15,37.59 49.55,37.95 49.55,40.12 JP1.6 | 49.28,15.24 49.28,12.45 49.78,11.94 49.78,5.08 49.55,4.85 49.55,2.18 49.15,1.78 48.59,1.78 48.59,1.72 JP2.6 | 49.28,15.24 50.67,15.24 | R37.2 51.47,15.66 51.05,15.24 50.67,15.24 | 50.67,15.24 v50.67,15.62
SDA  (via drill 0.25)
  Top 0.203: 44.45,13.59 44.06,13.59 | U6.7 44.39,13.64 44.45,13.59 | 44.45,13.59 44.96,13.59 45.59,12.95 v45.59,12.7 | U4.29 36.16,17.49 35.56,16.89 v35.56,14.86
  Route15 0.203: v45.59,12.7 43.18,15.11 38.86,15.11 | 38.86,15.11 35.81,15.11 v35.56,14.86 | TP19.TP 9.27,14.35 9.78,14.86 31.24,14.86 31.75,14.35 31.75,13.72 32.64,12.83 38.86,12.83 38.86,15.11
  Bottom 0.203: R38.R1_1 38.08,15.34 37.57,14.83 35.66,14.83 v35.56,14.86
SDA_IN  (via drill 0.25)
  Top 0.203: U9.20 49.93,12.05 49.66,12.32 46.99,12.32 46.1,13.21 46.1,13.59 v45.97,13.59 45.72,13.59 44.96,14.35 44.45,14.35 U6.6 | J2.2 67.64,20.46 67.28,20.83 64.74,20.83 64.36,20.45 64.36,17.02 63.98,16.64 50.55,16.64 | v47.37,13.46 47.24,13.72 47.24,14.99 47.75,15.49 49.4,15.49 50.55,16.64 | 50.55,16.64 50.55,17.45 50.6,17.53 50.6,19.68 v50.29,19.68
  Bottom 0.203: JP2.4 47.55,2.72 47.55,6.81 48.64,8 48.64,11.05 47.37,12.32 v47.37,13.46 47.37,13.59 v45.97,13.59 45.47,13.59 45.09,13.97 45.09,14.48 44.58,14.99 44.58,20.45 43.69,21.34 43.69,33.27 43.94,33.53 43.94,36.32 45.34,37.72 47.37,37.72 47.55,37.9 47.55,40.08 46.53,41.1 46.53,41.13 JP1.4
  Bottom 0.254: v50.29,19.68 50.8,19.68 51.18,19.3 51.18,18.41 R39.2
SHARE_CLK  (via drill 0.25)
  Top 0.203: U4.18 30.66,18.72 30.48,18.54 v28.57,18.54 | v38.73,19.18 38.73,16.51 39.65,16.51 R15.R3_1 40.49,16.49 40.64,16.64 40.64,19.43 40.89,19.68 41.53,19.68 43.56,17.65 43.56,16.13 43.81,15.88 45.21,15.88 45.97,15.11 v45.97,14.86
  Bottom 0.203: 45.47,14.86 45.47,14.35 45.59,14.22 47.62,14.22 48.01,13.84 48.01,12.32 49.02,11.3 49.02,7.49 48.53,7 48.53,3.72 JP2.5 | v45.97,14.86 45.47,14.86 | 45.47,14.86 44.96,15.37 44.96,20.45 45.34,20.83 45.34,32.64 46.86,32.64 48.64,34.42 48.64,35.43 | 48.64,35.43 48.64,37.59 48.51,37.72 48.51,39.12 48.53,39.13 JP1.5 | 48.64,35.43 TP5.TP | v28.57,18.54 36.2,18.54 36.83,19.18 v38.73,19.18
SHORT  (via drill 0.25)
  Top 0.406: v13.59,24 13.59,21.84 13.59,21.64 13.59,21.46 SW2.SW1
  Route15 0.203: v13.59,24 13.59,23.75 13.46,23.62 8,23.62 6.6,22.23 6.6,18.16 9.53,15.24 32.64,15.24 33.66,14.22 33.66,13.59 33.91,13.34 36.07,13.34 36.32,13.59 v36.32,14.1
  Bottom 0.203: v36.32,14.1 36.32,13.46 36.45,13.34 37.21,13.34 37.47,13.08 37.47,11.68 37.34,11.56 35.69,11.56 35.69,9.78 35.31,9.4 35.31,7.75 35.16,7.61 Q7.1 | 13.59,25.27 R43.2
  Bottom 0.406: 13.59,25.27 v13.59,24 13.59,22.86 R41.2
SW2  (via drill 0.25)
  Top 0.203: v30.99,12.83 NB8.1
  Bottom 0.203: v30.99,12.83 30.99,11.18 30.86,11.05 29.97,11.05 R31.R2_1
SW3
  Top 0.203: NB8.2 33.66,12.32 33.66,12.57 L5.1
  pour Top (no thermals): 32.26,13.34 36.45,13.34 36.45,11.68 32.51,11.68 32.26,12.06
SW4  (via drill 0.25)
  Top 0.203: v15.62,12.83 NB7.1
  Bottom 0.203: v15.62,12.83 15.62,11.18 15.49,11.05 14.61,11.05 R32.R2_1
SW5
  Top 0.203: NB7.2 18.29,12.32 18.29,12.57 L4.1
  pour Top (no thermals): 16.89,13.34 21.08,13.34 21.08,11.68 17.14,11.68 16.89,12.06
SW7  (via drill 0.25)
  Top 0.203: NB3.1 v23.37,33.53
  Bottom 0.203: v23.37,33.53 23.37,35.18 23.5,35.31 24.38,35.31 R51.R2_1
SW8
  Top 0.203: NB3.2 20.7,34.04 20.7,33.78 L1.1
  pour Top (no thermals): 22.1,33.02 17.91,33.02 17.91,34.67 21.84,34.67 22.1,34.29
SW9  (via drill 0.25)
  Top 0.203: NB4.1 v38.73,33.53
  Bottom 0.203: v38.73,33.53 38.73,35.18 38.86,35.31 39.75,35.31 R50.R2_1
SW10
  Top 0.203: NB4.2 36.07,34.04 36.06,33.78 L2.1
  pour Top (no thermals): 37.47,33.02 33.27,33.02 33.27,34.67 37.21,34.67 37.47,34.29
SW_LTC3604
  Top 0.203: 47.44,25.37 C12.1
  pour Top (no thermals): 43.81,28.83 46.23,28.83 47.12,27.94 47.12,24.89 48.64,24.89 48.64,28.96 47.62,28.96 47.62,32 43.81,32
TEMP_CH0
  Top 0.203: C25.1 13.04,9.27 12.57,9.27 12.56,9.29 12.56,12.08 12.45,12.19 12.45,12.83 Q3.2 12.45,13.13 12.45,13.46 12.57,13.59 TP15.1 14.48,16 22.23,16 22.48,16.26 22.48,21.72 22.73,21.97 24.26,21.97 24.51,21.72 24.51,19.56 24.77,19.3 27.81,19.3 28.19,19.68 28.19,20.32 28.5,20.63 U4.15
TEMP_CH1
  Top 0.203: C26.1 28.41,9.27 27.94,9.27 27.93,9.29 27.93,12.08 27.81,12.19 27.81,12.83 Q4.2 27.81,13.13 27.81,13.46 27.94,13.59 TP17.1 27.94,18.8 28.7,19.56 28.7,20.07 28.76,20.13 U4.16
TEMP_CH2  (via drill 0.25)
  Top 0.203: C7.1 25.95,37.08 26.42,37.08 26.43,37.07 26.43,34.27 26.54,34.16 26.54,33.53 Q1.2 26.54,33.22 26.54,32.89 26.42,32.77 TP9.1 26.42,32 26.92,31.5 34.16,31.5 34.67,30.99 37.47,30.99 37.85,30.61 v37.85,29.46 | U4.27 35.16,17.93 v35.31,17.78
  Route15 0.203: v37.85,29.46 37.85,28.57 38.48,27.94 41.4,27.94 41.66,27.69 41.66,24.13 41.15,23.62 35.43,23.62 34.92,23.11 34.92,18.03 35.18,17.78 v35.31,17.78
TEMP_CH3
  Top 0.203: C8.1 41.31,37.08 41.78,37.08 41.8,37.07 41.8,34.27 41.91,34.16 41.91,33.53 Q2.2 41.91,33.22 41.91,32.89 41.78,32.77 TP11.1 42.55,31.5 42.55,30.1 42.04,29.59 42.04,28.07 42.55,27.56 42.55,20.83 42.34,20.63 U4.34
UNUSED1
  Route15 0.203: JP1.9 52.55,38.39 52.83,38.1 59.05,38.1 59.69,38.73 67.44,38.73 68.2,37.97 68.2,22.23 66.55,20.57 66.55,19.18 66.09,18.73 64.57,18.73 64.39,18.54 64.39,10.41 62.23,8.26 62.23,6.99 61.85,6.6 53.21,6.6 52.58,5.97 52.58,3.75 JP2.9
UNUSED2  (via drill 0.25)
  Top 0.203: v53.54,5.21 53.54,2.74 JP2.10
  Route15 0.203: JP1.10 52.58,41.13 52.58,41.91 53.09,42.42 57.66,42.42 58.42,41.66 58.42,40.51 59.69,39.24 67.94,39.24 68.71,38.48 68.71,9.27 68.07,8.64 63.37,8.64 62.87,8.13 62.87,6.86 62.1,6.1 53.98,6.1 53.54,5.66 v53.54,5.21
VDD  (via drill 0.25)
  Top 0.203: v40.13,7.75 41.27,7.75 41.27,7.11 41.31,7.24 R19.2 | v24.77,7.75 25.91,7.75 25.91,7.11 25.95,7.24 R18.2 | v14.22,38.61 13.08,38.61 13.08,39.24 13.04,39.12 R5.2 | v29.59,38.61 28.45,38.61 28.45,39.24 28.41,39.12 R6.2
  Top 0.254: C14.2 27.51,23.13 U4.10
  Top 0.406: 27.18,23.5 C14.2 | 27.18,23.5 26.92,23.5 | 27.18,23.5 27.18,24.26 26.92,24.51 v25.15,24.51 | SW2.SW2 19.56,21.46 v19.56,22.73 | R10.2 46.74,20.7 48.39,19.05 TP14.TP
  Bottom 0.203: R29.2 40.13,5.97 | R30.2 24.77,5.97 | 14.22,40.39 R53.2 | 29.59,40.39 R52.2
  Bottom 0.406: 40.13,5.97 v40.13,7.75 | 24.77,5.97 v24.77,7.75 | v14.22,38.61 14.22,40.39 | v29.59,38.61 29.59,40.39
  other vias: 41.02,4.45 25.65,4.45 13.34,41.91 28.7,41.91 67.06,25.53 64.49,24.23 67.06,26.8 67.06,24.26
  pour Top (no thermals): 35.81,10.67 36.45,10.67 36.45,9.14 36.7,8.89 37.47,8.89 37.72,9.14 37.72,10.67 42.29,10.67 42.29,6.86 40.77,6.86 40.51,6.6 40.51,5.21 40.77,4.95 41.53,4.95 41.53,4.06 39.5,4.06 39.5,6.99 38.35,8.13 36.58,8.13 35.81,8.89
  pour Top (no thermals): 20.45,10.67 21.08,10.67 21.08,9.14 21.34,8.89 22.1,8.89 22.35,9.14 22.35,10.67 26.92,10.67 26.92,6.86 25.4,6.86 25.15,6.6 25.15,5.21 25.4,4.95 26.16,4.95 26.16,4.06 24.13,4.06 24.13,6.99 22.99,8.13 21.21,8.13 20.45,8.89
  pour Top (no thermals): 18.54,35.69 17.91,35.69 17.91,37.21 17.65,37.47 16.89,37.47 16.64,37.21 16.64,35.69 12.06,35.69 12.06,39.5 13.59,39.5 13.84,39.75 13.84,41.15 13.59,41.4 12.83,41.4 12.83,42.29 14.86,42.29 14.86,39.37 16,38.23 17.78,38.23 18.54,37.47
  pour Top (no thermals): 33.91,35.69 33.27,35.69 33.27,37.21 33.02,37.47 32.26,37.47 32,37.21 32,35.69 27.43,35.69 27.43,39.5 28.96,39.5 29.21,39.75 29.21,41.15 28.96,41.4 28.19,41.4 28.19,42.29 30.23,42.29 30.23,39.37 31.37,38.23 33.15,38.23 33.91,37.47
  pour Route15 (no thermals): 0.89,45.59 0.89,2.29 2.41,0.76 68.93,0.76 68.93,45.59
  pour Top (no thermals): 64.14,27.18 67.69,27.18 67.69,23.88 64.14,23.88
  pour Bottom (no thermals): 64.14,27.18 67.69,27.18 67.69,23.88 64.14,23.88
VDD_OR
  Top 0.203: U5.16 U5.15 57.68,26.44 57.78,26.54 60.07,26.54 60.2,26.42 60.2,25.22 U5.10 U5.9 | R7.1 NB5.1
  pour Top (no thermals): 57.02,27.18 63.75,27.18 63.75,23.88 62.36,23.88 61.59,24.64 60.2,24.64 60.2,26.16 57.66,26.16 57.66,24.64 57.02,24.64
VFB  (via drill 0.25)
  Top 0.203: U8.5 37.08,10.79 36.7,11.18 34.16,11.18 34.04,11.3 33.02,11.3 32.89,11.18 31.75,11.18 | 31.75,11.18 30.86,11.18 30.73,11.05 30.73,10.16 31.88,9.02 31.88,5.88 | 31.75,5.84 31.88,5.84 | 31.75,5.84 31.62,5.84 | 31.88,5.88 31.75,5.84 | 31.75,11.18 v31.75,11.56 | R22.2 31.88,5.88
  Top 0.254: 31.79,5.97 R22.2
  Top 0.406: 31.79,5.97 C35.2 31.75,4.45 31.75,3.3 R26.1
  Bottom 0.203: v31.75,11.56 31.75,11.18 32.64,11.18 32.64,10.67 32.38,10.67 R34.1
VFB1  (via drill 0.25)
  Top 0.203: U7.5 21.72,10.79 21.34,11.18 18.8,11.18 18.67,11.3 17.65,11.3 17.53,11.18 16.38,11.18 | 16.38,11.18 15.49,11.18 15.37,11.05 15.37,10.16 16.51,9.02 16.51,5.88 | 16.38,5.84 16.51,5.84 | 16.38,5.84 16.26,5.84 | 16.51,5.88 16.38,5.84 | 16.38,11.18 v16.38,11.56 | R21.2 16.51,5.88
  Top 0.254: 16.42,5.97 R21.2
  Top 0.406: 16.42,5.97 C33.2 16.38,4.45 16.38,3.3 R25.1
  Bottom 0.203: v16.38,11.56 16.38,11.18 17.27,11.18 17.27,10.67 17.02,10.67 R36.1
VFB2  (via drill 0.25)
  Top 0.203: U1.5 17.27,35.56 17.65,35.18 20.19,35.18 20.32,35.05 21.34,35.05 21.46,35.18 22.61,35.18 | 22.61,35.18 23.5,35.18 23.62,35.31 23.62,36.2 22.48,37.34 22.48,40.47 | 22.61,40.51 22.48,40.51 | 22.61,40.51 22.73,40.51 | 22.48,40.47 22.61,40.51 | 22.61,35.18 v22.61,34.8 | 22.48,40.47 R3.2
  Top 0.254: R3.2 22.57,40.39
  Top 0.406: 22.57,40.39 C1.2 22.61,41.91 22.61,43.05 R1.1
  Bottom 0.203: v22.61,34.8 22.61,35.18 21.72,35.18 21.72,35.69 21.97,35.69 R48.1
VFB3  (via drill 0.25)
  Top 0.203: U2.5 32.64,35.56 33.02,35.18 35.56,35.18 35.69,35.05 36.7,35.05 36.83,35.18 37.97,35.18 | 37.97,35.18 38.86,35.18 38.99,35.31 38.99,36.2 37.85,37.34 37.85,40.47 | 37.97,40.51 37.85,40.51 | 37.97,40.51 38.1,40.51 | 37.85,40.47 37.97,40.51 | 37.97,35.18 v37.97,34.8 | 37.85,40.47 R4.2
  Top 0.254: R4.2 37.93,40.39
  Top 0.406: 37.93,40.39 C3.2 37.97,41.91 37.97,43.05 R2.1
  Bottom 0.203: v37.97,34.8 37.97,35.18 37.08,35.18 37.08,35.69 37.34,35.69 R46.1
VIN_SNS_CAP  (via drill 0.25)
  Top 0.203: v36.96,29.46 36.83,29.46 36.66,29.29 U4.51
  Bottom 0.203: v36.96,29.46 36.83,29.46 36.7,29.34 36.7,27.3 36.58,27.27 C49.2
VOUT_CH0
  Top 0.203: L4.2 NB9.2
  Top 0.254: R25.2 18.12,3.3 C33.1 21.59,4.45 TP21.TP
  pour Top (no thermals): 16.89,10.54 19.94,10.54 19.94,8.64 20.95,7.62 22.73,7.62 23.62,6.73 23.62,3.94 21.97,2.29 17.65,2.29 17.65,4.95 19.18,4.95 20.07,5.84 20.07,6.48 19.43,7.11 16.89,7.11
  pour Bottom (no thermals): 15.88,2.29 15.88,3.81 16.64,4.57 18.8,4.57 20.07,5.84 20.07,9.14 20.57,9.65 20.57,11.3 22.1,11.3 22.99,10.41 26.54,10.41 26.8,10.16 26.8,8.51 24.26,8.51 23.88,8.13 23.88,4.19 21.97,2.29
VOUT_CH1
  Top 0.203: L5.2 NB10.2
  Top 0.254: R26.2 33.49,3.3 C35.1 36.96,4.45 TP22.TP
  pour Top (no thermals): 32.26,10.54 35.31,10.54 35.31,8.64 36.32,7.62 38.1,7.62 38.99,6.73 38.99,3.94 37.34,2.29 33.02,2.29 33.02,4.95 34.54,4.95 35.43,5.84 35.43,6.48 34.8,7.11 32.26,7.11
  pour Bottom (no thermals): 31.24,2.29 31.24,3.81 32,4.57 34.16,4.57 35.43,5.84 35.43,9.14 35.94,9.65 35.94,11.3 37.47,11.3 38.35,10.41 41.91,10.41 42.16,10.16 42.16,8.51 39.62,8.51 39.24,8.13 39.24,4.19 37.34,2.29
VOUT_CH2
  Top 0.203: NB1.2 L1.2
  Top 0.254: R1.2 20.87,43.05 C1.1 17.4,41.91 TP3.TP
  pour Top (no thermals): 22.1,35.81 19.05,35.81 19.05,37.72 18.03,38.73 16.26,38.73 15.37,39.62 15.37,42.42 17.02,44.07 21.34,44.07 21.34,41.4 19.81,41.4 18.92,40.51 18.92,39.88 19.56,39.24 22.1,39.24
  pour Bottom (no thermals): 23.11,44.07 23.11,42.55 22.35,41.78 20.19,41.78 18.92,40.51 18.92,37.21 18.41,36.7 18.41,35.05 16.89,35.05 16,35.94 12.45,35.94 12.19,36.2 12.19,37.85 14.73,37.85 15.11,38.23 15.11,42.16 17.02,44.07
VOUT_CH3
  Top 0.203: NB2.2 L2.2
  Top 0.254: R2.2 36.23,43.05 C3.1 32.77,41.91 TP4.TP
  pour Top (no thermals): 37.47,35.81 34.42,35.81 34.42,37.72 33.4,38.73 31.62,38.73 30.73,39.62 30.73,42.42 32.38,44.07 36.7,44.07 36.7,41.4 35.18,41.4 34.29,40.51 34.29,39.88 34.92,39.24 37.47,39.24
  pour Bottom (no thermals): 38.48,44.07 38.48,42.55 37.72,41.78 35.56,41.78 34.29,40.51 34.29,37.21 33.78,36.7 33.78,35.05 32.26,35.05 31.37,35.94 27.81,35.94 27.56,36.2 27.56,37.85 30.1,37.85 30.48,38.23 30.48,42.16 32.38,44.07
VREF
  Bottom 0.406: U11.6 51.8,22.54 R40.2 51.94,22.35 51.94,24 C47.2
VSNS_CH0  (via drill 0.25)
  Top 0.203: U4.1 28.76,27.63 28.32,28.07 v28.07,28.07
  Route15 0.203: v26.16,16.64 26.54,17.02 26.54,27.18 27.43,28.07 v28.07,28.07
  Bottom 0.203: 21.08,12.45 R35.2 | C44.2 19.43,12.45 | TP27.1 19.43,14.73 19.94,15.24 25.78,15.24 26.16,15.62 v26.16,16.64
  Bottom 0.406: TP27.1 19.43,12.45 21.08,12.45
VSNS_CH1  (via drill 0.25)
  Top 0.203: v28.07,28.96 28.45,29.34 30.35,29.34 30.66,29.03 U4.63
  Route15 0.203: v25.02,17.65 25.78,18.41 25.78,28.57 26.8,29.59 27.81,29.59 28.07,29.34 v28.07,28.96
  Bottom 0.203: 36.45,12.45 R33.2 | 34.8,12.45 C43.2 | TP23.1 33.78,14.1 32.64,15.24 29.46,15.24 27.05,17.65 v25.02,17.65
  Bottom 0.406: TP23.1 34.8,12.45 36.45,12.45
VSNS_CH2
  Top 0.203: U4.61 31.62,28.45 31.62,28.96 31.41,29.17 31.41,30.32 31.11,30.61 30.99,30.61 21.97,30.61 20.32,32.26 TP38.1
  Bottom 0.203: 17.91,33.91 R49.2 | 19.56,33.91 C55.2
  Bottom 0.406: TP38.1 19.56,33.91 17.91,33.91
VSNS_CH3
  Top 0.203: U4.49 37.72,28.45 38.1,28.45 38.61,28.96 38.61,30.73 37.85,31.5 35.18,31.5 34.8,31.88 TP34.1
  Bottom 0.203: 33.27,33.91 R47.2 | 34.8,33.91 C54.2
  Bottom 0.406: TP34.1 34.8,33.91 33.27,33.91

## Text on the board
tPlace: CH2 2.5V | CH3 3.3V | GND | INSTALL CONNECTORS | ON TOP SIDE | F | E | M | A | L | E | GND | 6-14V | 0.3A | 0.3A | FAULT | - | + | SHARE_CLK | CONTROL | ALERT | FAULT | RESET | ALERT | SCL | LTC2975CUP | SHORT | +5V | SDA | DEMO CIRCUIT 2022A | RUN | OFF | 0.3A | 0.3A | CONTROL | CH0 1.5V | CH1 1.8V | M | A | L | E | GND
bPlace: CH2 2.5V | CH3 3.3V | REV 1 | ISP | RUN | VS | DAC | ISP | ISN | TEMP | RUN | VS | DAC | ISN | TMP | LTC CONFIDENTIAL | FOR CUSTOMER USE | ONLY | VS | TMP | ISN | ISP | DAC | VS | RUN | TEMP | ISN | ISP | DAC | FLT | RUN | HI | LO | A2 | A1 | A0 | 1 | CH0 1.5V | CH1 1.8V
tStop: LTC2975CUP | POWER SYSTEM | MANAGER | (408) 432-1900 | www.linear.com
bStop: MANAGER | POWER SYSTEM | LTC2975CUP | (408) 432-1900 | www.linear.com
d_FabDrawing: 1.825" | DRILL TABLE | 0.00" | 2.755" | 0.00" | SHOWN FROM TOP SIDE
